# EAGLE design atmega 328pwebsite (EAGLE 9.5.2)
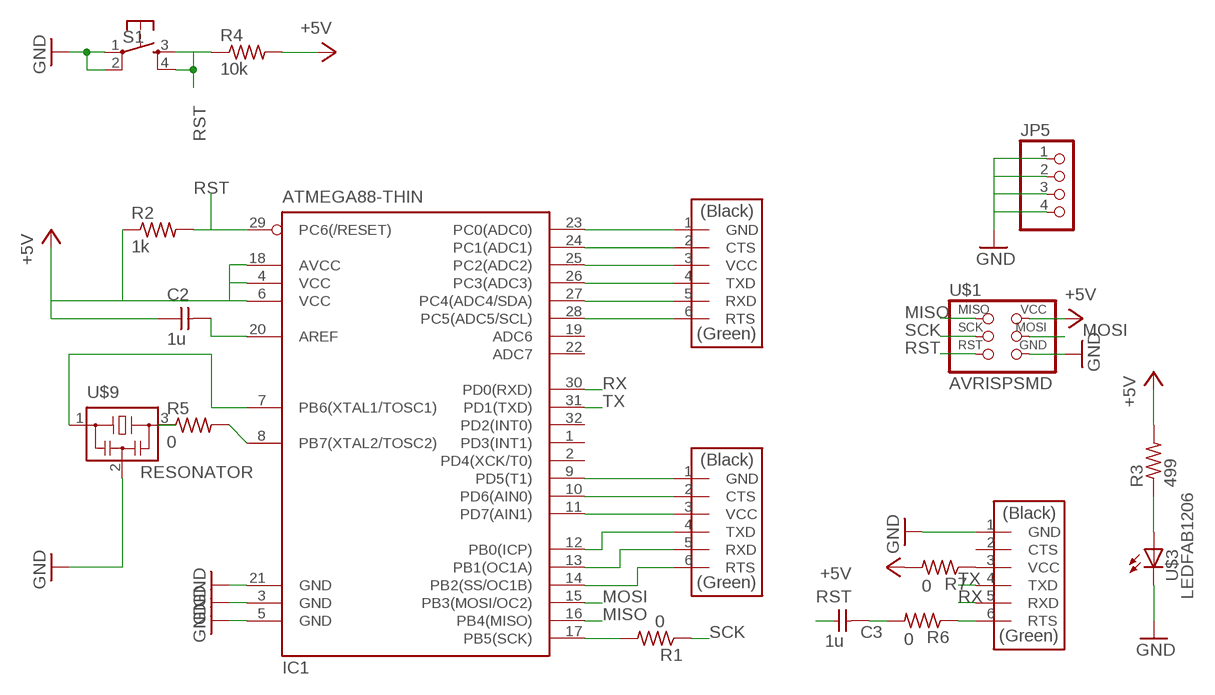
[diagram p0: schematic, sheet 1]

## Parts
C2  1u  CAP-UNPOLARIZEDFAB  [C1206FAB]
C3  1u  CAP-UNPOLARIZEDFAB  [C1206FAB]
IC1  ATMEGA88-THIN  [TQFP32-08THIN]
JP5  PINHD-1X4  [1X04]
R1  0  RES-US1206FAB  [R1206FAB]
R2  1k  RES-US1206FAB  [R1206FAB]
R3  499  RES-US1206FAB  [R1206FAB]
R4  10k  RES-US1206FAB  [R1206FAB]
R5  0  RES-US1206FAB  [R1206FAB]
R6  0  RES-US1206FAB  [R1206FAB]
R7  0  RES-US1206FAB  [R1206FAB]
S1  6MM_SWITCH6MM_SWITCH  [6MM_SWITCH]
U$1  AVRISPSMD  [2X03SMD]
U$2  FTDI-SMD-HEADER  [1X06SMD]
U$3  LEDFAB1206  [LED1206FAB]
U$5  CONN_06_FTDI-SMD-HEADER  [1X06SMD]
U$9  RESONATOR  [EFOBM]
U$10  CONN_06_FTDI-SMD-HEADER  [1X06SMD]

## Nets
+5V: C2.1 IC1.4(VCC) IC1.6(VCC) IC1.18(AVCC) R2.1 R3.2 R4.2 R7.2 U$1.2(VCC)
GND: IC1.3(GND) IC1.5(GND) IC1.21(GND) JP5.1 JP5.2 JP5.3 JP5.4 S1.1(P) S1.2(P1) U$1.6(GND) U$2.1(GND) U$3.2(C) U$9.2
MISO: IC1.16(PB4(MISO)) U$1.1(MISO)
MOSI: IC1.15(PB3(MOSI/OC2)) U$1.4(MOSI)
N$1: IC1.7(PB6(XTAL1/TOSC1)) U$9.1
N$2: IC1.8(PB7(XTAL2/TOSC2)) R5.2
N$3: R5.1 U$9.3
N$4: R3.1 U$3.1(A)
N$5: C2.2 IC1.20(AREF)
N$6: C3.2 R6.2
N$7: IC1.23(PC0(ADC0)) U$10.1(GND)
N$8: IC1.24(PC1(ADC1)) U$10.2(CTS)
N$9: IC1.25(PC2(ADC2)) U$10.3(VCC)
N$10: IC1.26(PC3(ADC3)) U$10.4(TXD)
N$11: IC1.27(PC4(ADC4/SDA)) U$10.5(RXD)
N$12: IC1.28(PC5(ADC5/SCL)) U$10.6(RTS)
N$13: IC1.9(PD5(T1)) U$5.1(GND)
N$14: IC1.10(PD6(AIN0)) U$5.2(CTS)
N$15: IC1.11(PD7(AIN1)) U$5.3(VCC)
N$16: IC1.12(PB0(ICP)) U$5.4(TXD)
N$17: IC1.13(PB1(OC1A)) U$5.5(RXD)
N$18: IC1.14(PB2(SS/OC1B)) U$5.6(RTS)
N$19: R6.1 U$2.6(RTS)
N$20: R7.1 U$2.3(VCC)
RST: C3.1 IC1.29(PC6(/RESET)) R2.2 R4.1 S1.3(S) S1.4(S1) U$1.5(RST)
RX: IC1.30(PD0(RXD)) U$2.5(RXD)
SCK: IC1.17(PB5(SCK)) R1.1 R1.2 U$1.3(SCK)
TX: IC1.31(PD1(TXD)) U$2.4(TXD)
Unconnected: IC1.1(PD3(INT1)) IC1.2(PD4(XCK/T0)) IC1.19(ADC6) IC1.22(ADC7) IC1.32(PD2(INT0)) U$2.2(CTS)

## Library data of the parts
C2 C3 = fab:CAP-UNPOLARIZED
IC1 = fab:ATMEGA88-THIN
JP5 = pinhead:PINHD-1X4: PIN HEADER
R1-R7 = fab:RES-US: Resistor (US Symbol)
S1 = fab:6MM_SWITCH: OMRON SWITCH
U$1 = fab:AVRISP
U$2 = fab:FTDI-SMD-HEADER
U$3 = fab:LED: LED
U$5 U$10 = fab:CONN_06_FTDI-SMD-HEADER
U$9 = fab:RESONATOR

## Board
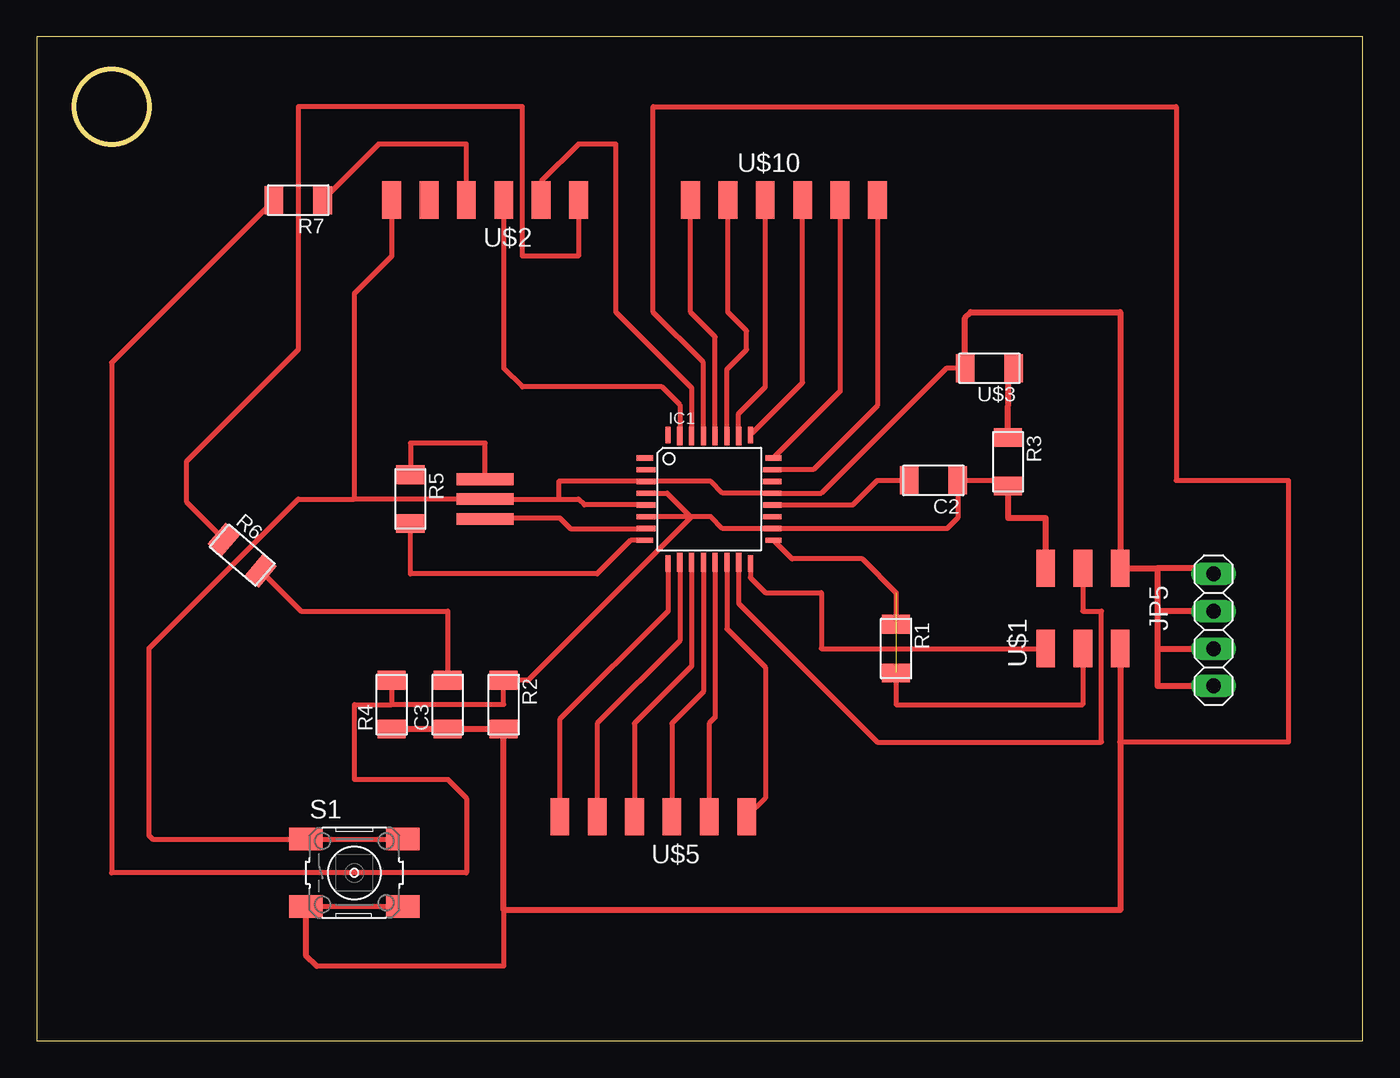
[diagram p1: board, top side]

Size 90.15 x 68.25 mm. Coordinates in mm from the lower left corner, seen from the top.
Outline: 0,0 90.15,0 90.15,68.25 0,68.25 0,0
Outline: circle at 5.08,63.5 radius 2.54
Copper layers (1*16): Top 0.035mm / dielectric 1.5mm / Bottom 0.035mm
Design rules "default *": minimum track width 14mil, minimum drill 0.35mm, track to track 16mil, track to pad 16mil, pad to pad 16mil, via to via 16mil, smd to smd 16mil, copper to edge 16mil, drill to drill 16mil, minimum pad ring 10mil, minimum via ring 8mil, stop-mask expansion 4mil, vias tented up to drill 0mil, thermal gap 10mil

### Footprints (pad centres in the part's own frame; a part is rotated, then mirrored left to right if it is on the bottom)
C1206FAB = smd 1.27 x 1.905: 1 -1.651,0; 2 1.651,0
TQFP32-08THIN = smd 1.118 x 0.356: 1 -4.369,2.8; 8 -4.369,-2.8; 17 4.369,-2.8; 24 4.369,2.8 | smd 1.27 x 0.356: 2 -4.293,2; 3 -4.293,1.2; 4 -4.293,0.4; 5 -4.293,-0.4; 6 -4.293,-1.2; 7 -4.293,-2; 18 4.293,-2; 19 4.293,-1.2; 20 4.293,-0.4; 21 4.293,0.4; 22 4.293,1.2; 23 4.293,2 | smd 0.356 x 1.118: 9 -2.8,-4.369; 16 2.8,-4.369; 25 2.8,4.369; 32 -2.8,4.369 | smd 0.356 x 1.27: 10 -2,-4.293; 14 1.2,-4.293; 15 2,-4.293; 26 2,4.293; 27 1.2,4.293; 31 -2,4.293 | smd 0.35 x 1.27: 11 -1.2,-4.293; 12 -0.4,-4.293; 13 0.4,-4.293; 28 0.4,4.293; 29 -0.4,4.293; 30 -1.2,4.293
1X04 = drill 1.016 long: 1 -3.81,0; 2 -1.27,0; 3 1.27,0; 4 3.81,0
R1206FAB = smd 1.27 x 1.905: 1 -1.651,0; 2 1.651,0
6MM_SWITCH = smd 2.286 x 1.524: 1 -3.302,2.286; 2 3.302,2.286; 3 -3.302,-2.286; 4 3.302,-2.286
2X03SMD = smd 2.54 x 1.27: 1 -2.54,2.54; 2 2.92,2.54; 3 -2.54,0; 4 2.92,0; 5 -2.54,-2.54; 6 2.92,-2.54
1X06SMD = smd 2.54 x 1.27: 1 0,6.35; 2 0,3.81; 3 0,1.27; 4 0,-1.27; 5 0,-3.81; 6 0,-6.35
LED1206FAB = smd 1.27 x 1.905: 1 -1.651,0; 2 1.651,0
EFOBM = smd 0.8 x 3.9: 1 -1.35,0; 2 0,0; 3 1.35,0

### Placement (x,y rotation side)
C2  60.96,38.1 180 top
C3  27.94,22.86 90 top
IC1  45.72,36.83 0 top
JP5  80.01,27.94 90 top
R1  58.42,26.67 270 top
R2  31.75,22.86 270 top
R3  66.04,39.37 270 top
R4  24.13,22.86 90 top
R5  25.4,36.83 270 top
R6  13.97,33.02 319.4 top
R7  17.78,57.15 180 top
S1  21.59,11.43 0 top
U$1  71.12,29.21 90 top
U$2  30.48,57.15 90 top
U$3  64.77,45.72 180 top
U$5  41.91,15.24 90 top
U$9  30.48,36.83 90 top
U$10  50.8,57.15 270 top

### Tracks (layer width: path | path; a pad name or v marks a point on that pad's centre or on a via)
+5V
  Top 0.356: 44.45,35.63 45.83,35.63 46.63,34.83 IC1.18 61.88,34.83 62.61,35.56 C2.1 65.66,38.1 | 44.45,35.63 IC1.6 | IC1.4 42.85,37.23 44.45,35.63 | R4.2 24.13,22.86 | 24.13,22.86 31.75,22.86 R2.1 33.4,24.51 44.45,35.56 44.45,35.63 | R7.2 5.08,46.1 5.08,11.43 29.21,11.43 29.21,16.51 27.94,17.78 21.59,17.78 21.59,22.86 24.13,22.86
  Top 0.406: U$1.2 68.58,35.56 66.04,35.56 R3.2 65.66,38.1
GND
  Top 0.356: U$2.1 24.13,53.34 21.59,50.8 21.59,36.83 | 21.59,36.83 U$9.2 35.56,36.83 | U$3.2 61.83,45.72 53.34,37.23 IC1.21 46.63,37.23 45.83,38.03 IC1.3 35.49,38.03 35.49,36.9 35.56,36.83 | 35.56,36.83 36.83,36.83 37.23,36.43 IC1.5 | S1.2 S1.1 7.87,13.72 7.62,13.97 7.62,26.67 17.78,36.83 21.59,36.83
  Top 0.406: 76.2,32.13 U$1.6 73.66,49.53 63.5,49.53 63.12,49.15 U$3.2 | 76.2,32.13 79.63,32.13 JP5.4 | 76.2,32.13 76.2,29.21 | JP5.3 76.2,29.21 | 76.2,29.21 76.2,26.67 | 76.2,26.67 JP5.2 | 76.2,26.67 76.2,24.13 JP5.1
MISO
  Top 0.356: IC1.16 48.52,31.49 49.53,30.48 53.34,30.48 53.34,26.67 U$1.1
MOSI
  Top 0.356: U$1.4 71.12,29.21 72.39,29.21 72.39,20.32 57.15,20.32 47.72,29.75 IC1.15
N$1
  Top 0.356: IC1.7 36.29,34.83 35.56,35.56 30.56,35.56 U$9.1
N$2
  Top 0.356: R5.2 25.4,31.75 38.1,31.75 40.38,34.03 IC1.8
N$3
  Top 0.356: U$9.3 30.48,40.64 25.4,40.64 R5.1
N$4
  Top 0.406: U$3.1 66.04,45.34 66.04,43.18 | R3.1 66.04,43.18 | 66.04,43.18
N$5
  Top 0.356: IC1.20 55.48,36.43 57.15,38.1 C2.2
N$6
  Top 0.356: R6.2 17.96,29.21 27.94,29.21 C3.2
N$7
  Top 0.356: U$10.1 57.15,43.18 53.34,39.37 52.8,38.83 IC1.23
N$8
  Top 0.356: U$10.2 54.61,44.15 IC1.24
N$9
  Top 0.356: IC1.25 52.07,44.75 U$10.3
N$10
  Top 0.356: IC1.26 47.72,42.64 49.53,44.45 U$10.4
N$11
  Top 0.356: IC1.27 46.92,45.65 48.26,46.99 48.26,48.26 46.99,49.53 46.99,53.34 U$10.5
  Top 0.406: U$10.5 46.92,57.08
N$12
  Top 0.356: IC1.28 46.12,47.86 44.45,49.53 U$10.6
N$13
  Top 0.356: IC1.9 42.92,29.21 35.56,21.85 U$5.1
N$14
  Top 0.356: IC1.10 43.72,27.21 38.1,21.59 U$5.2
N$15
  Top 0.356: IC1.11 44.52,25.47 40.64,21.59 U$5.3
N$16
  Top 0.356: IC1.12 45.32,23.73 43.18,21.59 U$5.4
N$17
  Top 0.356: IC1.13 46.12,21.99 45.72,21.59 U$5.5
N$18
  Top 0.356: IC1.14 46.92,28.01 49.53,25.4 49.53,16.51 U$5.6
N$19
  Top 0.356: U$2.6 36.83,53.34 33.02,53.34 33.02,63.5 17.78,63.5 17.78,46.99 10.16,39.37 10.16,36.65 R6.1
N$20
  Top 0.356: U$2.3 29.21,60.96 23.24,60.96 R7.1
RST
  Top 0.356: 73.66,20.32 85.09,20.32 85.09,38.1 77.47,38.1 77.47,63.5 41.91,63.5 41.91,49.53 45.32,46.12 IC1.29 | 31.75,8.89 31.75,5.08 19.05,5.08 | S1.3 S1.4
  Top 0.406: U$1.5 73.66,20.32 73.66,8.89 31.75,8.89 R2.2 C3.1 R4.1 | S1.3 18.29,5.84 19.05,5.08
RX
  Top 0.356: U$2.5 34.29,58.42 36.83,60.96 39.37,60.96 39.37,49.53 44.52,44.38 IC1.30
SCK  (1 unrouted)
  Top 0.356: IC1.17 51.36,32.76 56.14,32.76 58.42,30.48 R1.1 | U$1.3 71.12,22.86 58.42,22.86 R1.2
TX
  Top 0.356: IC1.31 43.72,43.23 42.5,44.45 33.02,44.45 31.75,45.72 U$2.4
